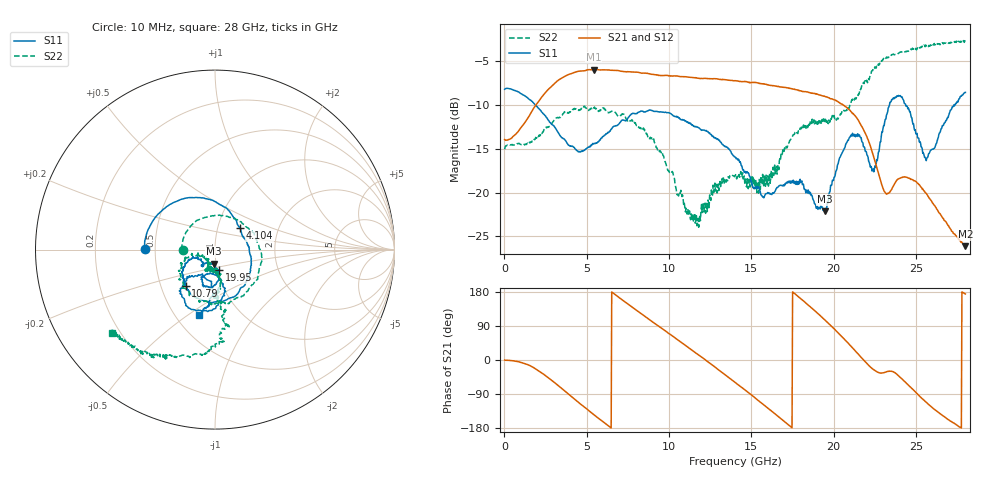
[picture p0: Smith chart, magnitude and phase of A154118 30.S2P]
!  2-Port S-parameters saved by WinCal
! VAR MeasName=S-Parameters (CALIBRATED_DATA) read from VNA (N5230A)
! VAR MeasDate=2015-9-10 14:36:38
! VAR NAME=A154118 30
! VAR FILENAME=A154118 30.S2P
! VAR DATE=2015-9-10 14:36:38
! VAR PHYS_PORTS=1,2
# Hz S DB R 50
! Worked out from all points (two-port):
!   801 points, 10 MHz to 28 GHz, reference 50 ohm
!   highest |S21| = -5.94 dB at 5.433 GHz (marker M1); lowest = -26.1 dB at 28 GHz (marker M2)
!   |S21| within 3 dB of the highest: 2.33 GHz to 19.3 GHz (16.97 GHz wide, 157 % of centre)
!   lowest |S11| = -22.1 dB at 19.46 GHz (marker M3), VSWR 1.17, Z = 48.7 - j7.62 ohm
!   |S11| at or under -10 dB: 1.877 GHz to 23.39 GHz (21.51 GHz wide, 170 % of centre); 24.38 GHz to 27.3 GHz (2.919 GHz wide, 11.3 % of centre); 27.30493 GHz to 27.36122 GHz (56.29 MHz wide, 0.206 % of centre)
!   |S22| runs from -24.0 to -2.6 dB; largest |S21 - S12| = 0.0085
!   S11 on the Smith chart (normalised r, x): 10 MHz: 0.44, +0.00; 4.104 GHz: 1.28, +0.32; 10.79 GHz: 0.67, -0.29; 19.95 GHz: 1.02, -0.24; 28 GHz: 0.65, -0.55
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1e7  -8.20 179.7  -13.94 -0.2  -14.00 -0.1  -15.05 180.0
1.794362e9  -9.80 116.4  -10.30 -20.7  -10.32 -20.5  -13.93 63.5
3.053912e9  -12.53 73.0  -7.51 -60.0  -7.51 -60.0  -11.67 -6.6
4.103538e9  -14.70 40.3  -6.38 -97.6  -6.38 -97.7  -10.65 -53.2
4.698325e9  -15.32 24.5  -6.12 -118.9  -6.11 -119.1  -10.40 -73.2
5.433062e9  -14.40 2.2  -5.94 -144.4  -5.94 -144.4  -10.35 -93.8
7.0075e9  -12.02 -46.7  -6.10 163.3  -6.08 163.4  -11.30 -127.5
9.351662e9  -10.77 -104.7  -6.62 89.5  -6.55 89.4  -15.10 -164.1
1.078615e10  -11.69 -128.7  -6.76 45.1  -6.70 44.5  -20.45 -161.2
1.173081e10  -12.49 -139.4  -6.94 15.0  -6.88 14.4  -23.46 -129.6
1.4005e10  -15.93 -158.3  -7.24 -58.9  -7.23 -59.4  -18.13 -114.0
1.529954e10  -19.34 -154.8  -7.43 -102.6  -7.38 -103.2  -18.96 -95.0
1.662906e10  -19.35 -129.0  -7.85 -148.8  -7.84 -149.5  -16.84 -78.4
1.869332e10  -20.37 -125.7  -8.63 136.1  -8.68 135.6  -11.62 -88.7
1.946305e10  -22.14 -95.6  -9.01 105.7  -9.04 105.2  -12.05 -90.1
1.995288e10  -18.62 -79.0  -9.36 85.3  -9.34 84.8  -11.45 -88.0
2.110746e10  -13.56 -95.8  -10.87 34.0  -10.86 32.7  -9.38 -82.5
2.243699e10  -17.63 -94.9  -15.95 -25.9  -16.02 -26.3  -5.77 -84.3
2.334666e10  -10.21 -86.5  -20.07 -30.1  -20.03 -30.4  -4.56 -99.4
2.446626e10  -10.15 -128.2  -18.28 -63.2  -18.22 -64.1  -3.85 -113.5
2.562085e10  -16.35 -117.2  -20.07 -111.6  -20.12 -111.6  -3.22 -119.5
2.8e10  -8.56 -103.8  -26.11 174.2  -26.12 173.4  -2.63 -140.9
